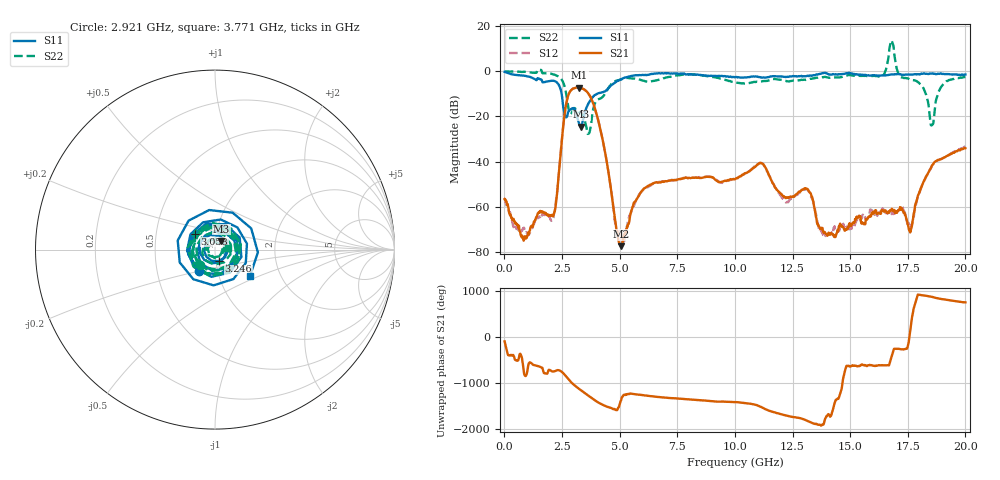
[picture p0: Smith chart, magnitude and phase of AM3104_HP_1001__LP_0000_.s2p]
!Created with skrf (http://scikit-rf.org).
# Hz S RI R 50.0
!freq ReS11 ImS11 ReS21 ImS21 ReS12 ImS12 ReS22 ImS22
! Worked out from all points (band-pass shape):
!   1601 points, 10 MHz to 20 GHz, reference 50 ohm
!   highest |S21| = -7.18 dB at 3.246 GHz (marker M1); lowest = -77.5 dB at 5.07 GHz (marker M2)
!   |S21| within 3 dB of the highest: 2.789 GHz to 3.663 GHz (873.8 MHz wide, 27.1 % of centre)
!   lowest |S11| = -24.5 dB at 3.333 GHz (marker M3), VSWR 1.13, Z = 53.3 + j5.15 ohm
!   |S11| at or under -10 dB: 2.483 GHz to 4.026 GHz (1.542 GHz wide, 47.4 % of centre)
!   |S22| runs from -27.8 to 13.7 dB; largest |S21 - S12| = 0.023
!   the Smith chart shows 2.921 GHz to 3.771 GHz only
!   S11 on the Smith chart (normalised r, x): 2.921 GHz: 0.81, -0.20; 3.058 GHz: 0.79, +0.14; 3.246 GHz: 1.03, -0.13; 3.771 GHz: 1.40, -0.44
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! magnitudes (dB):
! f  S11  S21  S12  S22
! 10 MHz  -0.3  -56.6  -56.1  0.0
! 847.1 MHz  -2.0  -74.9  -69.3  -0.2
! 2.084 GHz  -4.1  -63.7  -65.8  -1.2
! 2.646 GHz  -19.9  -16.7  -16.6  -8.2
! 2.921 GHz  -16.5  -8.1  -8.2  -18.4
! 3.058 GHz  -16.9  -7.4  -7.4  -16.4
! 3.246 GHz  -23.4  -7.2  -7.3  -18.2
! 3.333 GHz  -24.5  -7.4  -7.5  -18.6
! 3.346 GHz  -24.4  -7.5  -7.5  -18.7
! 3.771 GHz  -12.2  -12.1  -12.2  -22.8
! 5.07 GHz  -3.5  -77.5  -73.6  -3.5
! 6.682 GHz  -0.9  -49.2  -49.2  -3.8
! 10.01 GHz  -2.6  -47.9  -47.5  -4.9
! 11.14 GHz  -2.7  -40.7  -40.8  -4.5
! 12.18 GHz  -2.5  -55.8  -57.7  -4.2
! 13.34 GHz  -1.9  -55.6  -56.3  -3.3
! 13.9 GHz  -0.7  -71.4  -72.5  -2.5
! 16.68 GHz  -1.5  -62.3  -62.6  7.2
! 17.61 GHz  -1.4  -71.2  -69.5  -3.6
! 18.54 GHz  -0.9  -42.0  -42.2  -23.9
! 19 GHz  -1.2  -38.7  -38.6  -6.2
! 20 GHz  -1.4  -34.1  -33.3  -2.5
